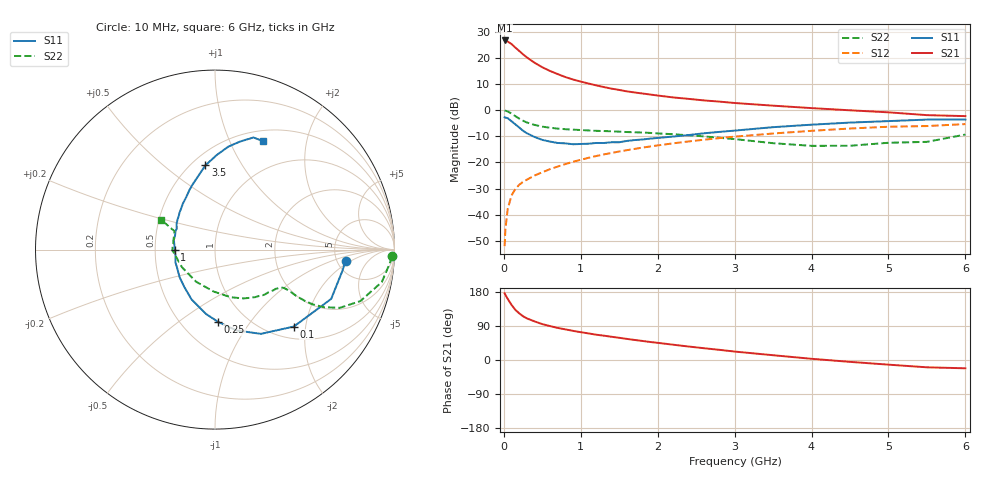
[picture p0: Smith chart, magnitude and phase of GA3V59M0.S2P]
! Infineon Technologies  Discrete & RF Semiconductors
! BF775
! Si NPN RF Bipolar Junction Transistor in SOT23
! VCE = 3.5 V  IC = 9 mA
! Common Emitter S-Parameters:  May  1996
# GHz  S  MA  R  50
!  f  S11  S21  S12  S22
! GHz  MAG  ANG  MAG  ANG  MAG  ANG  MAG  ANG
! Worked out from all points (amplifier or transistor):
!   36 points, 10 MHz to 6 GHz, reference 50 ohm
!   highest |S21| = 26.7 dB at 10 MHz (marker M1)
!   |S21| within 3 dB of that: start of sweep to 160.3 MHz
!   unconditionally stable (mu >= 1): 604.6 MHz to 3.289 GHz
!   at 250 MHz: K = 0.66, MSG = 24.4 dB, |S12| = -27.4 dB
!   at 1.4 GHz: K = 1.11, MAG = 10.3 dB, |S12| = -16.4 dB
!   at 6 GHz: K = 0.95, MSG = 1.5 dB, |S12| = -5.3 dB
!   S11 on the Smith chart (normalised r, x): 10 MHz: 5.98, -1.56; 100 MHz: 1.25, -1.72; 250 MHz: 0.74, -0.71; 1 GHz: 0.63, +0.00; 3.5 GHz: 0.58, +0.71; 6 GHz: 0.63, +1.35
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0.01  0.7297 -4.8  21.56 176.0  0.0025 91.0  0.9853 -2.2
0.02  0.7198 -9.4  21.22 172.0  0.0052 82.6  0.9764 -4.6
0.05  0.7032 -23.0  20.55 161.3  0.0128 78.3  0.9468 -11.0
0.1  0.6137 -44.3  18.4 145.4  0.0234 70.6  0.8593 -19.5
0.15  0.5347 -61.4  15.73 132.3  0.0311 65.1  0.7675 -25.0
0.2  0.4656 -75.2  13.58 123.1  0.0374 62.4  0.6887 -27.8
0.25  0.4034 -87.5  11.69 115.4  0.0426 60.9  0.627 -29.2
0.3  0.3614 -98.1  10.19 109.8  0.0468 61.1  0.5807 -29.7
0.4  0.3067 -115.2  8.068 101.8  0.0563 61.5  0.522 -29.7
0.5  0.2701 -129.1  6.615 94.7  0.0648 62.6  0.4842 -29.2
0.6  0.2504 -141.8  5.628 89.5  0.0744 63.3  0.4609 -29.0
0.7  0.2358 -152.5  4.899 84.7  0.0834 63.5  0.4435 -29.1
0.8  0.2316 -162.4  4.297 80.8  0.093 63.6  0.4321 -29.4
1  0.2255 180.0  3.522 73.4  0.1123 63.6  0.4167 -30.7
1.1  0.2281 173.3  3.235 70.2  0.1225 63.4  0.4091 -32.0
1.3  0.2354 161.1  2.767 64.2  0.1424 62.4  0.3986 -34.2
1.6  0.2579 146.0  2.287 55.7  0.1719 60.2  0.3813 -38.5
2.2  0.3127 124.9  1.754 40.4  0.2318 54.8  0.3468 -49.8
3.5  0.4726 96.5  1.219 12.6  0.3576 39.4  0.2334 -92.0
4.5  0.5786 82.6  0.994 -4.9  0.4454 26.2  0.2084 -151.6
5.5  0.6603 71.1  0.803 -19.3  0.4966 11.4  0.2475 155.6
6  0.6613 65.9  0.769 -21.9  0.5416 7.4  0.3414 151.1
